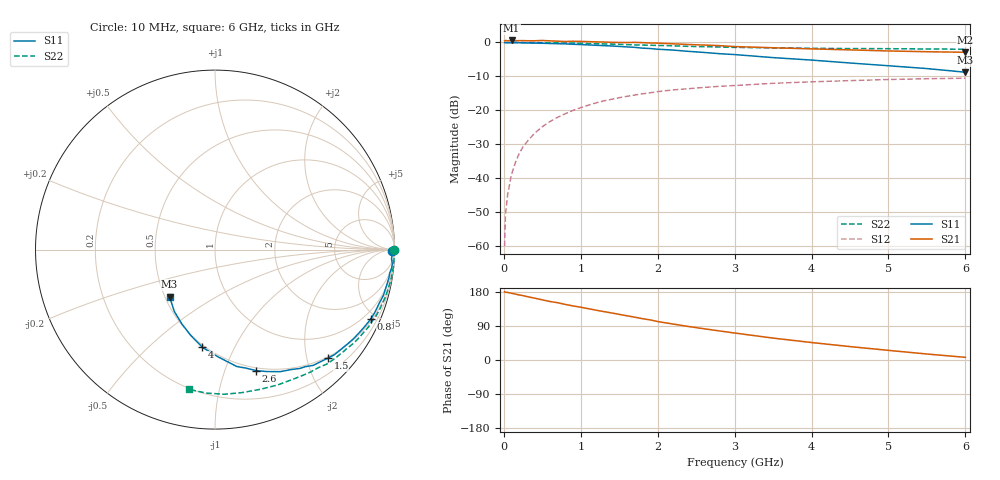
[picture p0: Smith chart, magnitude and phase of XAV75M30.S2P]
! SIEMENS Discrete & RF Semiconductors
! BFY180
! Si NPN RF Bipolar Junction Transistor in MICRO-X
! VCE = 0.75 V  IC = 0.3 mA
! Common Emitter S-Parameters:  May  1997
# GHz  S  MA  R  50
!  f  S11  S21  S12  S22
! GHz  MAG  ANG  MAG  ANG  MAG  ANG  MAG  ANG
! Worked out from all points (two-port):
!   36 points, 10 MHz to 6 GHz, reference 50 ohm
!   highest |S21| = 0.57 dB at 100 MHz (marker M1); lowest = -2.9 dB at 6 GHz (marker M2)
!   |S21| within 3 dB of the highest: start of sweep to 4.854 GHz
!   lowest |S11| = -8.8 dB at 6 GHz (marker M3), VSWR 2.14, Z = 26.5 - j15.9 ohm
!   |S11| at or under -10 dB: nowhere
!   |S22| runs from -2.0 to 0.0 dB; largest |S21 - S12| = 1.1
!   S11 on the Smith chart (normalised r, x): 10 MHz: open; 800 MHz: 0.58, -4.64; 1.5 GHz: 0.47, -2.40; 2.6 GHz: 0.47, -1.29; 4 GHz: 0.48, -0.76; 6 GHz: 0.53, -0.32
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0.01  0.9873 -0.3  1.055 180.0  0.001 90.8  0.9999 -0.1
0.02  0.9859 -0.7  1.067 178.9  0.0028 91.9  0.9995 -0.4
0.05  0.9873 -1.5  1.056 178.3  0.0058 86.3  0.9986 -1.1
0.1  0.9849 -3.0  1.068 176.0  0.0114 88.3  0.9988 -2.3
0.15  0.9914 -4.6  1.06 174.0  0.017 85.7  0.9986 -3.4
0.2  0.9894 -6.0  1.061 171.6  0.0231 84.8  0.997 -4.5
0.25  0.9819 -7.8  1.062 169.9  0.0291 84.0  0.9994 -5.7
0.4  0.9761 -12.2  1.057 163.2  0.0461 80.3  0.9954 -9.0
0.5  0.9724 -15.2  1.067 158.8  0.0573 77.3  0.9914 -11.3
0.6  0.9626 -18.1  1.054 154.3  0.0684 74.6  0.9881 -13.5
0.8  0.9505 -24.0  1.03 146.6  0.0893 69.9  0.9794 -18.0
1.1  0.9182 -32.6  1.026 135.4  0.1192 62.4  0.9624 -24.5
1.5  0.8724 -43.9  0.998 120.4  0.1536 53.1  0.9362 -32.8
1.8  0.8233 -52.4  0.992 109.1  0.1749 47.3  0.9138 -38.4
2.2  0.771 -61.9  0.953 94.9  0.1998 39.1  0.8913 -45.7
2.6  0.712 -71.2  0.915 82.5  0.2173 32.7  0.865 -52.1
3  0.6621 -79.5  0.868 71.2  0.2316 26.5  0.8449 -58.2
3.5  0.597 -88.5  0.834 57.8  0.2499 20.1  0.831 -65.2
4  0.549 -97.3  0.803 46.1  0.2627 13.8  0.8181 -72.2
4.5  0.4974 -105.7  0.776 35.4  0.2737 8.0  0.8109 -79.3
5.5  0.4118 -123.5  0.729 15.8  0.2917 -3.1  0.8008 -93.6
6  0.3639 -134.1  0.715 7.0  0.2972 -8.8  0.7922 -100.7
